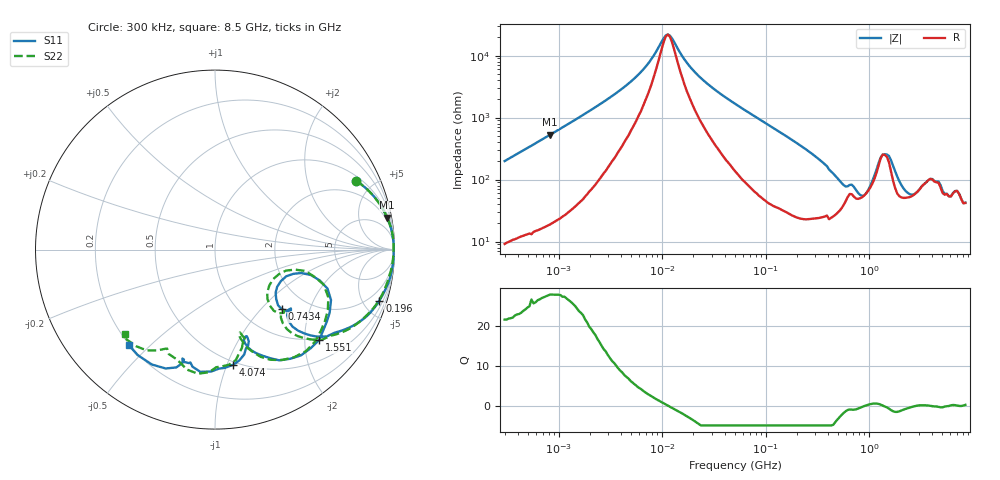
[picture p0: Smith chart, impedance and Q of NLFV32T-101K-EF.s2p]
! S-parameter Generated by TDK Corporation
! Copyright(C) 2015 TDK Corporation.
! All Rights Reserved.
! TDK P/N: NLFV32T-101K-EF (Inductors)
! Property: L=100uH at 796kHz
! Size(LxWxT): 3.2x2.5x2.2mm, 0.126x0.098x0.087inches
! Model Type: s2p (Touchstone File Format Version 1.0)
! Frequency: DC=Yes Start=0.3MHz Stop=8500MHz 225points Log-sweep
! Note:
! Model Generated on Jun. 23, 2015
! Hash(MD5):
! Port Assignments:
!  1 ---@@@--- 2
! Applicable Conditions:
!  Temperature = 25 degC
!  DC Bias Current = 0 A
!  Small Signal Operation
! Terms and conditions regarding TDK Simulation Models
! (1)This simulation model is being provided solely for informational purposes. Please refer to the specifications of the products in terms of detailed characteristics of such products.
! (2)In no event shall TDK Corporation of any of its subsidiaries be liable for any loss or damage arising, directly or indirectly,
!  From any information contained in this simulation model, including, but not limited to loss or damages arising from any inaccuracies, omissions or errors in connection with such information.
! (3)Any and all copyrights on this simulation model are owned by TDK Corporation.
!  Duplication or redistribution of this simulation model without prior written permission from TDK Corporation is prohibited.
! (4)This simulation model is subject to any modification or change without any prior notice.
! (5)Neither TDK Corporation nor any of its subsidiaries shall make any warranty, express or implied,
!  Including but not limited to the correctness, implied warranties of merchantability and fitness for a particular purpose with respect to this simulation models.
! (6)The use of this simulation model shall be deemed to have consented to the terms and conditions hereof.
# MHz S MA R 50
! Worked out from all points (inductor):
!   224 points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, 300 kHz to 8.5 GHz, reference 50 ohm
!   read as one part in series: L = 104 uH near 314.1 kHz
!   highest Q = 28 at 824.8 kHz (marker M1), where L = 102 uH
!   self-resonance near 10.82 MHz
!   S11 on the Smith chart (normalised r, x): 300 kHz: 1.21, +4.00; 196 MHz: 0.92, -6.46; 743.4 MHz: 1.49, -1.32; 1.551 GHz: 0.96, -2.35; 4.074 GHz: 0.48, -1.05; 8.5 GHz: 0.20, -0.43
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0.3  0.8764 25.9  0.442 -61.4  0.4469 -61.6  0.8753 25.9
0.8248242  0.9759 10.5  0.185 -77.5  0.1858 -77.8  0.9761 10.5
1.72111  0.9919 5.0  0.08987 -82.5  0.09021 -82.8  0.9926 5.0
5.431819  0.9956 1.2  0.02292 -78.3  0.02296 -78.7  0.9956 1.0
9.430415  0.9955 0.1  0.00684 -48.7  0.006838 -49.1  0.9955 -0.1
11.86747  0.9955 -0.3  0.004738 15.4  0.004734 15.0  0.9953 -0.5
20.60362  0.9956 -1.4  0.01826 74.2  0.01827 74.0  0.995 -1.6
51.67171  0.9946 -4.4  0.06088 80.8  0.06092 80.5  0.991 -4.8
195.9978  0.9588 -17.3  0.2387 68.6  0.2389 68.4  0.9508 -18.4
283.1228  0.9122 -25.1  0.3452 59.0  0.3456 58.8  0.8994 -26.6
448.3627  0.7425 -40.7  0.5481 37.1  0.5484 36.7  0.7289 -43.3
743.4462  0.4993 -41.7  0.6123 6.9  0.6123 6.5  0.4727 -46.1
935.5712  0.4068 -25.6  0.6145 -14.4  0.6147 -15.0  0.363 -27.0
1124.446  0.5522 -14.9  0.4722 -32.7  0.4722 -32.9  0.5167 -13.3
1351.452  0.729 -28.8  0.2681 -23.2  0.2684 -23.5  0.7129 -28.1
1551.304  0.7685 -40.9  0.2765 0.5  0.2768 -0.1  0.7575 -42.4
1780.71  0.7382 -55.5  0.4112 6.5  0.4113 6.1  0.7191 -58.9
2240.89  0.5971 -70.1  0.5408 -13.9  0.5413 -14.1  0.5504 -72.8
3091.568  0.5235 -69.7  0.4992 -42.9  0.4995 -43.0  0.4992 -72.5
4073.536  0.6493 -80.9  0.3669 -48.9  0.369 -49.9  0.6461 -83.1
7072.242  0.691 -108.2  0.3154 -76.1  0.3168 -76.8  0.6787 -124.2
8500  0.7166 -132.1  0.3032 -89.2  0.3027 -88.4  0.6858 -136.8
